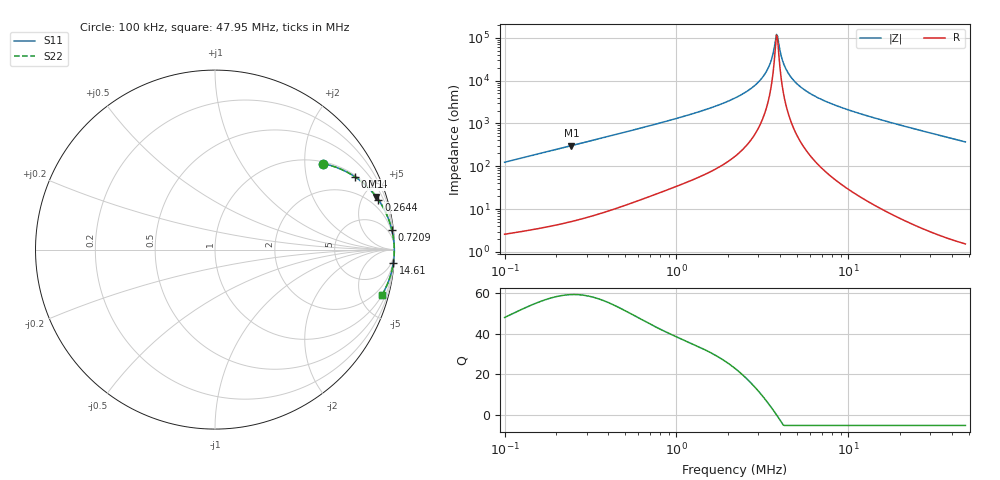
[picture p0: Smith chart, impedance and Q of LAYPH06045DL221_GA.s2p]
! LAYPH06045DL221_GA  S-PARAMETER MODEL  ( General Type )
! Model Generated by TAIYO YUDEN Corporation (http://www.ty-top.com)
! Version 2.0
! TAIYO YUDEN Control No. 180914NI43SB-FBB
! Copyright(c) 2018 TAIYO YUDEN CO.,LTD. All Rights Reserved.
! Product Description (link to TY-COMPAS)
! https://ds.yuden.co.jp/TYCOMPAS/or/detail?pn=LAYPH06045DL221MGA&u=M
! Products Name : Inductors
! Characteristics :
!  Inductance : 220 uH , SRF(min) : -Hz , DC Resistance(max) : 0.804 Ohm
!  Rated Current : Saturation :0.44 A , Temp Rise : 0.36 A (25 degC)
!  Case Size : 6.3 x 6.0 / 0.248 x 0.236 [mm/inch] , Thickness : 4.5 / 0.177 [mm/inch]
!  (Conditions: Temperature = 25 degC , DC Bias Current/Voltage = 0A / 0V)
! External Node Assignments :
!  1  o---GGG---o  2
! GND o---------o GND
! Frequency Range : 0.1MHz  -  47.953651MHz  [ 402 STEP ]
# MHz S RI R 50
! Freq[MHz].  S11 Real  S11 Imag  S21 Real  S21 Imag  S12 Real  S12 Imag  S22 Real  S22 Imag
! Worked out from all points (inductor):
!   401 points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, 100 kHz to 47.95 MHz, reference 50 ohm
!   read as one part in series: L = 197 uH near 103.1 kHz
!   highest Q = 59.2 at 244.7 kHz (marker M1), where L = 197 uH
!   self-resonance near 3.817 MHz
!   S11 on the Smith chart (normalised r, x): 100 kHz: 1.05, +2.48; 154 kHz: 1.07, +3.81; 264.4 kHz: 1.11, +6.54; 720.9 kHz: 1, +18; 14.61 MHz: 1, -26; 47.95 MHz: 1.03, -7.41
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0.1  0.6042 0.4787  0.3958 -0.4787  0.3958 -0.4787  0.6042 0.4787
0.154049  0.7802 0.4052  0.2198 -0.4052  0.2198 -0.4052  0.7802 0.4052
0.244748  0.8977 0.2947  0.1023 -0.2947  0.1023 -0.2947  0.8977 0.2947
0.26438  0.9107 0.2768  0.0893 -0.2768  0.0893 -0.2768  0.9107 0.2768
0.281214  0.92 0.2629  0.08 -0.2629  0.08 -0.2629  0.92 0.2629
0.72088  0.9858 0.1076  0.0142 -0.1076  0.0142 -0.1076  0.9858 0.1076
0.790816  0.988 0.0977  0.012 -0.0977  0.012 -0.0977  0.988 0.0977
1.488879  0.9963 0.0468  0.00368 -0.0468  0.00368 -0.0468  0.9963 0.0468
2.223888  0.9983 0.0247  0.00171 -0.0247  0.00171 -0.0247  0.9983 0.0247
2.760207  0.9988 0.0145  0.00116 -0.0145  0.00116 -0.0145  0.9988 0.0145
3.220788  0.9991 0.00759  0.000935 -0.00759  0.000935 -0.00759  0.9991 0.00759
3.479144  0.9991 0.00422  0.000863 -0.00422  0.000863 -0.00422  0.9991 0.00422
3.816672  0.9992 0.000208  0.000812 -0.000208  0.000812 -0.000208  0.9992 0.000208
3.936306  0.9992 -0.00113  0.000803 0.00113  0.000803 0.00113  0.9992 -0.00113
4.186944  0.9992 -0.00381  0.000798 0.00381  0.000798 0.00381  0.9992 -0.00381
4.5228  0.9992 -0.00718  0.000815 0.00718  0.000815 0.00718  0.9992 -0.00718
5.117099  0.9991 -0.0127  0.000897 0.0127  0.000897 0.0127  0.9991 -0.0127
6.158125  0.9988 -0.0213  0.00116 0.0213  0.00116 0.0213  0.9988 -0.0213
8.647562  0.9978 -0.0392  0.00222 0.0392  0.00222 0.0392  0.9978 -0.0392
14.61381  0.9934 -0.0766  0.00658 0.0766  0.00658 0.0766  0.9934 -0.0766
17.31754  0.9907 -0.0924  0.00932 0.0924  0.00932 0.0924  0.9907 -0.0924
47.95365  0.9311 -0.2512  0.0689 0.2512  0.0689 0.2512  0.9311 -0.2512
